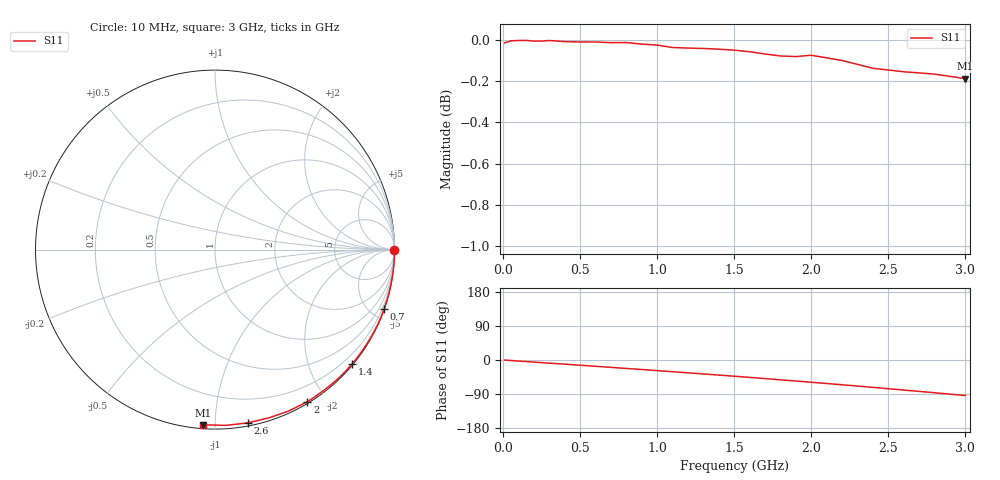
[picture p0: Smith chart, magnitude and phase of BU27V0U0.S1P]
! SIEMENS Small Signal Semiconductors
! BB833
! Si Tuning Diode in SOD323
! VR = 27 V
! S-Parameters:  April  1996
# GHz  S  MA  R  50
!  f  S11
! GHz  MAG  ANG
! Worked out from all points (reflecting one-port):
!   31 points, 10 MHz to 3 GHz, reference 50 ohm
!   lowest |S11| = -0.2 dB at 3 GHz (marker M1), VSWR 92.72, Z = 1.01 - j46.8 ohm
!   phase of S11 starts at -0 deg and turns -94 deg over the sweep
!   S11 on the Smith chart (normalised r, x): 10 MHz: open; 700 MHz: 0.03, -5.85; 1.4 GHz: 0.02, -2.76; 2 GHz: 0.02, -1.78; 2.6 GHz: 0.02, -1.21; 3 GHz: 0.02, -0.94
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0.01  0.9984 -0.1
0.02  0.9988 -0.5
0.05  0.9996 -1.3
0.1  0.9998 -2.8
0.15  0.9998 -4.1
0.3  0.9998 -8.3
0.4  0.9991 -11.0
0.5  0.999 -13.8
0.6  0.9989 -16.6
0.7  0.9986 -19.4
0.8  0.9986 -22.3
0.9  0.9978 -25.1
1  0.9972 -28.0
1.1  0.9959 -30.9
1.2  0.9956 -33.9
1.3  0.9953 -36.9
1.4  0.9949 -39.8
1.5  0.9944 -42.8
1.6  0.9935 -45.9
1.7  0.9922 -49.0
1.8  0.9912 -52.3
1.9  0.9908 -55.5
2  0.9916 -58.7
2.2  0.9887 -65.4
2.4  0.9843 -72.2
2.6  0.9824 -79.3
2.8  0.9811 -86.4
3  0.9787 -93.8
